| IBIS file stm32u5f9_5g9_lqfp100_dsi_smps.ibs
[IBIS ver] 4.2
[File name] stm32u5f9_5g9_lqfp100_dsi_smps.ibs
[File Rev] 1.0
[Date]  29-10-2024
[Source] Data Created at STMicroelectronics
[Notes]  File originated from ELDO simulations.
[Disclaimer]  This information is for modeling purpose only and is
   not guaranteed. The information is subject to change without
   notice.
[Copyright] Copyright 2024 STMicroelectronics Inc.
|   Component stm32u5f9_5g9_lqfp100_dsi_smps
[Component] stm32u5f9_5g9_lqfp100_dsi_smps
[Manufacturer] STMicroelectronics
[Package]
| variable   typ   min   max
R_pkg  0  NA  NA
L_pkg  0  NA  NA
C_pkg  0  NA  NA
[Pin]   signal_name   model_name
1  VBAT  power
2  PC13  io8_100m_ft_v33
3  PC14-OSC32_IN  io8_100m_ft
4  PC15-OSC32_OUT  io8_100m_ft
5  VDDDSI  nc
6  VDD11DSI  nc
7  DSI_D0P  nc
8  DSI_D0N  nc
9  VSSDSI  nc
10  DSI_CKP  nc
11  DSI_CKN  nc
12  VDD11DSI  nc
13  DSI_D1P  nc
14  DSI_D1N  nc
15  VSSDSI  nc
16  VDD  power
17  PH0-OSC_IN  io8_100m_ft
18  PH1-OSC_OUT  io8_100m_ft
19  NRST  nc
20  PC0  io8_100m_hslv_ft
21  PC1  io8_166m_hslv_i2c_ft
22  PC2  io8_100m_hslv_ft
23  PC3  io8_100m_hslv_ft
24  VSSA  nc
25  VDDA  nc
26  PA0  io8_100m_hslv_tamp_ft
27  PA1  io8_100m_hslv_tamp_ft
28  PA2  io8_100m_hslv_ft
29  PA3  io8_166m_hslv_ft
30  VSS  gnd
31  VDD  power
32  PA4  io8_100m_hslv_ft
33  PA5  io8_100m_ft
34  PA6  io8_100m_hslv_ft
35  PA7  io8_100m_hslv_ft
36  PB0  io8_100m_hslv_ft
37  PB1  io8_100m_hslv_ft
38  PB2  io8_100m_hslv_tamp_ft
39  PE7  io8_100m_hslv_ft
40  PE8  io8_100m_hslv_ft
41  PE9  io8_166m_hslv_ft
42  PE10  io8_166m_hslv_ft
43  VLXSMPS  nc
44  VDDSMPS  nc
45  VSSSMPS  nc
46  VDD11  nc
47  VSS  gnd
48  VDD  power
49  PB13  io8_100m_i2c_ft
50  PB14  io8_100m_hslv_ft
51  PB15  nc
52  PH9  io8_spi_ft
53  VSS  gnd
54  VDD  power
55  PH10  io8_spi_ft
56  PH11  io8_spi_ft
57  PH12  io8_spi_ft
58  PH13  io8_spi_ft
59  VSS  gnd
60  VDD  power
61  PH14  io8_spi_ft
62  PH15  io8_spi_ft
63  PI0  io8_spi_ft
64  PI1  io8_spi_ft
65  VSS  gnd
66  VDD  power
67  PI2  io8_spi_ft
68  PI3  io8_spi_ft
69  PA8  io8_166m_hslv_ft
70  PA9  io8_100m_usb_vbus_ft
71  PA10  io8_100m_usb_id
72  PA11  io8_100m_ft
73  PA12  io8_100m_ft
74  PA13  io8_100m_ft
75  VDDUSB  power
76  VDD  power
77  VSS  gnd
78  PA14  io8_100m_ft
79  PA15  nc
80  PC10  io8_100m_hslv_ft
81  PC11  io8_100m_hslv_ft
82  PC12  io8_166m_hslv_ft
83  PD0  io8_100m_hslv_ft
84  PD1  io8_100m_hslv_ft
85  PD2  io8_100m_hslv_ft
86  PD3  io8_166m_hslv_ft
87  PD4  io8_100m_hslv_ft
88  PD5  io8_100m_hslv_ft
89  VDD  power
90  PB3  io8_100m_hslv_ft
91  PB4  io8_100m_hslv_ft
92  PB5  io8_166m_hslv_ft
93  PB6  io8_100m_i2c_ft
94  PB7  io8_166m_hslv_i2c_ft
95  PH3-BOOT0  io8_100m_ft
96  PB8  io8_100m_hslv_ft
97  PB9  io8_100m_hslv_ft
98  VDD11  nc
99  VSS  gnd
100  VDD  power
[Package Model]   476-lqfp-14x14-100-dsi-smps-230223
[Pin Mapping]   pulldown_ref   pullup_ref   | Comment
1  nc  vsw
2  gndio  vddiom  | Depending on IO usage
| 2  gndio  vsw  | Depending on IO usage
3  gndio  vddiom  | Depending on IO usage
| 3  gndio  vsw  | Depending on IO usage
4  gndio  vddiom  | Depending on IO usage
| 4  gndio  vsw  | Depending on IO usage
5  nc  nc
6  nc  nc
7  nc  nc
8  nc  nc
9  nc  nc
10  nc  nc
11  nc  nc
12  nc  nc
13  nc  nc
14  nc  nc
15  nc  nc
16  nc  vddiom
17  gndio  vddiom
18  gndio  vddiom
19  nc  nc
20  gndio  vddiom
21  gndio  vddiom
22  gndio  vddiom
23  gndio  vddiom
24  nc  nc
25  nc  nc
26  gndio  vddiom
27  gndio  vddiom
28  gndio  vddiom
29  gndio  vddiom
30  gndio  nc
31  nc  vddiom
32  gndio  vddiom
33  gndio  vddiom
34  gndio  vddiom
35  gndio  vddiom
36  gndio  vddiom
37  gndio  vddiom
38  gndio  vddiom
39  gndio  vddiom
40  gndio  vddiom
41  gndio  vddiom
42  gndio  vddiom
43  nc  nc
44  nc  nc
45  nc  nc
46  nc  nc
47  gndio  nc
48  nc  vddiom
49  gndio  vddiom
50  gndio  vddiom
51  nc  nc
52  gndio  vddiom  | Depending on IO usage
| 52  gndio  vddhspi  | Depending on IO usage
53  gndio  nc
54  nc  vddhspi
55  gndio  vddiom
56  gndio  vddiom  | Depending on IO usage
| 56  gndio  vddhspi  | Depending on IO usage
57  gndio  vddiom  | Depending on IO usage
| 57  gndio  vddhspi  | Depending on IO usage
58  gndio  vddiom  | Depending on IO usage
| 58  gndio  vddhspi  | Depending on IO usage
59  gndio  nc
60  nc  vddhspi
61  gndio  vddiom  | Depending on IO usage
| 61  gndio  vddhspi  | Depending on IO usage
62  gndio  vddiom  | Depending on IO usage
| 62  gndio  vddhspi  | Depending on IO usage
63  gndio  vddiom  | Depending on IO usage
| 63  gndio  vddhspi  | Depending on IO usage
64  gndio  vddiom  | Depending on IO usage
| 64  gndio  vddhspi  | Depending on IO usage
65  gndio  nc
66  nc  vddhspi
67  gndio  vddiom  | Depending on IO usage
| 67  gndio  vddhspi  | Depending on IO usage
68  gndio  vddiom  | Depending on IO usage
| 68  gndio  vddhspi  | Depending on IO usage
69  gndio  vddiom
70  gndio  vddiom  | Depending on IO usage
| 70  gndio  vddusb  | Depending on IO usage
71  gndio  vddiom  | Depending on IO usage
| 71  gndio  vddusb  | Depending on IO usage
72  gndio  vddiom  | Depending on IO usage
| 72  gndio  vddusb  | Depending on IO usage
73  gndio  vddiom  | Depending on IO usage
| 73  gndio  vddusb  | Depending on IO usage
74  gndio  vddiom  | Depending on IO usage
| 74  gndio  vddusb  | Depending on IO usage
75  nc  vddusb
76  nc  vddiom
77  gndio  nc
78  gndio  vddiom
79  nc  nc
80  gndio  vddiom
81  gndio  vddiom
82  gndio  vddiom
83  gndio  vddiom
84  gndio  vddiom
85  gndio  vddiom
86  gndio  vddiom
87  gndio  vddiom
88  gndio  vddiom
89  nc  vddiom
90  gndio  vddiom
91  gndio  vddiom
92  gndio  vddiom
93  gndio  vddiom
94  gndio  vddiom
95  gndio  vddiom
96  gndio  vddiom
97  gndio  vddiom
98  nc  nc
99  gndio  nc
100  nc  vddiom
[Model Selector] io8_100m_ft
io8_100m_ft_hs_1v2  "IO8_FT 100MHz high speed @ 1.2V"
io8_100m_ft_fs_1v2  "IO8_FT 100MHz fast speed @ 1.2V"
io8_100m_ft_fs_pd_1v2  "IO8_FT 100MHz fast speed @ 1.2V pulldown"
io8_100m_ft_ms_1v2  "IO8_FT 100MHz med speed @ 1.2V"
io8_100m_ft_ms_pd_1v2  "IO8_FT 100MHz med speed @ 1.2V pulldown"
io8_100m_ft_ls_1v2  "IO8_FT 100MHz low speed @ 1.2V"
io8_100m_ft_ls_pd_1v2  "IO8_FT 100MHz low speed @ 1.2V pulldown"
io8_100m_ft_hs_1v8  "IO8_FT 100MHz high speed @ 1.8V"
io8_100m_ft_hs_pd_1v8  "IO8_FT 100MHz high speed @ 1.8V pulldown"
io8_100m_ft_fs_1v8  "IO8_FT 100MHz fast speed @ 1.8V"
io8_100m_ft_fs_pd_1v8  "IO8_FT 100MHz fast speed @ 1.8V pulldown"
io8_100m_ft_ms_1v8  "IO8_FT 100MHz med speed @ 1.8V"
io8_100m_ft_ms_pd_1v8  "IO8_FT 100MHz med speed @ 1.8V pulldown"
io8_100m_ft_ls_1v8  "IO8_FT 100MHz low speed @ 1.8V"
io8_100m_ft_ls_pd_1v8  "IO8_FT 100MHz low speed @ 1.8V pulldown"
io8_100m_ft_hs_3v3  "IO8_FT 100MHz high speed @ 3.3V"
io8_100m_ft_hs_pd_3v3  "IO8_FT 100MHz high speed @ 3.3V pulldown"
io8_100m_ft_fs_3v3  "IO8_FT 100MHz fast speed @ 3.3V"
io8_100m_ft_fs_pd_3v3  "IO8_FT 100MHz fast speed @ 3.3V pulldown"
io8_100m_ft_ms_3v3  "IO8_FT 100MHz med speed @ 3.3V"
io8_100m_ft_ms_pd_3v3  "IO8_FT 100MHz med speed @ 3.3V pulldown"
io8_100m_ft_ls_3v3  "IO8_FT 100MHz low speed @ 3.3V"
io8_100m_ft_ls_pd_3v3  "IO8_FT 100MHz low speed @ 3.3V pulldown"
[Model Selector] io8_100m_hslv_ft
io8_100m_ft_hs_1v2  "IO8_FT 100MHz high speed @ 1.2V"
io8_100m_ft_hs_pu_1v2  "IO8_FT 100MHz high speed @ 1.2V pullup"
io8_100m_ft_hs_pd_1v2  "IO8_FT 100MHz high speed @ 1.2V pulldown"
io8_100m_ft_fs_1v2  "IO8_FT 100MHz fast speed @ 1.2V"
io8_100m_ft_fs_pu_1v2  "IO8_FT 100MHz fast speed @ 1.2V pullup"
io8_100m_ft_fs_pd_1v2  "IO8_FT 100MHz fast speed @ 1.2V pulldown"
io8_100m_ft_ms_1v2  "IO8_FT 100MHz med speed @ 1.2V"
io8_100m_ft_ms_pu_1v2  "IO8_FT 100MHz med speed @ 1.2V pullup"
io8_100m_ft_ms_pd_1v2  "IO8_FT 100MHz med speed @ 1.2V pulldown"
io8_100m_ft_ls_1v2  "IO8_FT 100MHz low speed @ 1.2V"
io8_100m_ft_ls_pu_1v2  "IO8_FT 100MHz low speed @ 1.2V pullup"
io8_100m_ft_ls_pd_1v2  "IO8_FT 100MHz low speed @ 1.2V pulldown"
io8_100m_ft_hs_1v8  "IO8_FT 100MHz high speed @ 1.8V"
io8_100m_ft_hs_pu_1v8  "IO8_FT 100MHz high speed @ 1.8V pullup"
io8_100m_ft_hs_pd_1v8  "IO8_FT 100MHz high speed @ 1.8V pulldown"
io8_100m_ft_fs_1v8  "IO8_FT 100MHz fast speed @ 1.8V"
io8_100m_ft_fs_pu_1v8  "IO8_FT 100MHz fast speed @ 1.8V pullup"
io8_100m_ft_fs_pd_1v8  "IO8_FT 100MHz fast speed @ 1.8V pulldown"
io8_100m_ft_ms_1v8  "IO8_FT 100MHz med speed @ 1.8V"
io8_100m_ft_ms_pu_1v8  "IO8_FT 100MHz med speed @ 1.8V pullup"
io8_100m_ft_ms_pd_1v8  "IO8_FT 100MHz med speed @ 1.8V pulldown"
io8_100m_ft_ls_1v8  "IO8_FT 100MHz low speed @ 1.8V"
io8_100m_ft_ls_pu_1v8  "IO8_FT 100MHz low speed @ 1.8V pullup"
io8_100m_ft_ls_pd_1v8  "IO8_FT 100MHz low speed @ 1.8V pulldown"
io8_100m_ft_hs_3v3  "IO8_FT 100MHz high speed @ 3.3V"
io8_100m_ft_hs_pu_3v3  "IO8_FT 100MHz high speed @ 3.3V pullup"
io8_100m_ft_hs_pd_3v3  "IO8_FT 100MHz high speed @ 3.3V pulldown"
io8_100m_ft_fs_3v3  "IO8_FT 100MHz fast speed @ 3.3V"
io8_100m_ft_fs_pu_3v3  "IO8_FT 100MHz fast speed @ 3.3V pullup"
io8_100m_ft_fs_pd_3v3  "IO8_FT 100MHz fast speed @ 3.3V pulldown"
io8_100m_ft_ms_3v3  "IO8_FT 100MHz med speed @ 3.3V"
io8_100m_ft_ms_pu_3v3  "IO8_FT 100MHz med speed @ 3.3V pullup"
io8_100m_ft_ms_pd_3v3  "IO8_FT 100MHz med speed @ 3.3V pulldown"
io8_100m_ft_ls_3v3  "IO8_FT 100MHz low speed @ 3.3V"
io8_100m_ft_ls_pu_3v3  "IO8_FT 100MHz low speed @ 3.3V pullup"
io8_100m_ft_ls_pd_3v3  "IO8_FT 100MHz low speed @ 3.3V pulldown"
io8_100m_hslv_ft_hs_1v2  "IO8_FT 100MHz HSLV high speed @ 1.2V"
io8_100m_hslv_ft_hs_pu_1v2  "IO8_FT 100MHz HSLV high speed @ 1.2V pullup"
io8_100m_hslv_ft_hs_pd_1v2  "IO8_FT 100MHz HSLV high speed @ 1.2V pulldown"
io8_100m_hslv_ft_fs_1v2  "IO8_FT 100MHz HSLV fast speed @ 1.2V"
io8_100m_hslv_ft_fs_pu_1v2  "IO8_FT 100MHz HSLV fast speed @ 1.2V pullup"
io8_100m_hslv_ft_fs_pd_1v2  "IO8_FT 100MHz HSLV fast speed @ 1.2V pulldown"
io8_100m_hslv_ft_ms_1v2  "IO8_FT 100MHz HSLV med speed @ 1.2V"
io8_100m_hslv_ft_ms_pu_1v2  "IO8_FT 100MHz HSLV med speed @ 1.2V pullup"
io8_100m_hslv_ft_ms_pd_1v2  "IO8_FT 100MHz HSLV med speed @ 1.2V pulldown"
io8_100m_hslv_ft_ls_1v2  "IO8_FT 100MHz HSLV low speed @ 1.2V"
io8_100m_hslv_ft_ls_pu_1v2  "IO8_FT 100MHz HSLV low speed @ 1.2V pullup"
io8_100m_hslv_ft_ls_pd_1v2  "IO8_FT 100MHz HSLV low speed @ 1.2V pulldown"
io8_100m_hslv_ft_hs_1v8  "IO8_FT 100MHz HSLV high speed @ 1.8V"
io8_100m_hslv_ft_hs_pu_1v8  "IO8_FT 100MHz HSLV high speed @ 1.8V pullup"
io8_100m_hslv_ft_hs_pd_1v8  "IO8_FT 100MHz HSLV high speed @ 1.8V pulldown"
io8_100m_hslv_ft_fs_1v8  "IO8_FT 100MHz HSLV fast speed @ 1.8V"
io8_100m_hslv_ft_fs_pu_1v8  "IO8_FT 100MHz HSLV fast speed @ 1.8V pullup"
io8_100m_hslv_ft_fs_pd_1v8  "IO8_FT 100MHz HSLV fast speed @ 1.8V pulldown"
io8_100m_hslv_ft_ms_1v8  "IO8_FT 100MHz HSLV med speed @ 1.8V"
io8_100m_hslv_ft_ms_pu_1v8  "IO8_FT 100MHz HSLV med speed @ 1.8V pullup"
io8_100m_hslv_ft_ms_pd_1v8  "IO8_FT 100MHz HSLV med speed @ 1.8V pulldown"
io8_100m_hslv_ft_ls_1v8  "IO8_FT 100MHz HSLV low speed @ 1.8V"
io8_100m_hslv_ft_ls_pu_1v8  "IO8_FT 100MHz HSLV low speed @ 1.8V pullup"
io8_100m_hslv_ft_ls_pd_1v8  "IO8_FT 100MHz HSLV low speed @ 1.8V pulldown"
io8_100m_hslv_ft_hs_2v5  "IO8_FT 100MHz HSLV high speed @ 2.5V"
io8_100m_hslv_ft_hs_pu_2v5  "IO8_FT 100MHz HSLV high speed @ 2.5V pullup"
io8_100m_hslv_ft_hs_pd_2v5  "IO8_FT 100MHz HSLV high speed @ 2.5V pulldown"
io8_100m_hslv_ft_fs_2v5  "IO8_FT 100MHz HSLV fast speed @ 2.5V"
io8_100m_hslv_ft_fs_pu_2v5  "IO8_FT 100MHz HSLV fast speed @ 2.5V pullup"
io8_100m_hslv_ft_fs_pd_2v5  "IO8_FT 100MHz HSLV fast speed @ 2.5V pulldown"
io8_100m_hslv_ft_ms_2v5  "IO8_FT 100MHz HSLV med speed @ 2.5V"
io8_100m_hslv_ft_ms_pu_2v5  "IO8_FT 100MHz HSLV med speed @ 2.5V pullup"
io8_100m_hslv_ft_ms_pd_2v5  "IO8_FT 100MHz HSLV med speed @ 2.5V pulldown"
io8_100m_hslv_ft_ls_2v5  "IO8_FT 100MHz HSLV low speed @ 2.5V"
io8_100m_hslv_ft_ls_pu_2v5  "IO8_FT 100MHz HSLV low speed @ 2.5V pullup"
io8_100m_hslv_ft_ls_pd_2v5  "IO8_FT 100MHz HSLV low speed @ 2.5V pulldown"
[Model Selector] io8_100m_hslv_tamp_ft
io8_100m_ft_hs_1v2  "IO8_FT 100MHz high speed @ 1.2V"
io8_100m_ft_hs_pu_1v2  "IO8_FT 100MHz high speed @ 1.2V pullup"
io8_100m_ft_hs_pd_1v2  "IO8_FT 100MHz high speed @ 1.2V pulldown"
io8_100m_ft_fs_1v2  "IO8_FT 100MHz fast speed @ 1.2V"
io8_100m_ft_fs_pu_1v2  "IO8_FT 100MHz fast speed @ 1.2V pullup"
io8_100m_ft_fs_pd_1v2  "IO8_FT 100MHz fast speed @ 1.2V pulldown"
io8_100m_ft_ms_1v2  "IO8_FT 100MHz med speed @ 1.2V"
io8_100m_ft_ms_pu_1v2  "IO8_FT 100MHz med speed @ 1.2V pullup"
io8_100m_ft_ms_pd_1v2  "IO8_FT 100MHz med speed @ 1.2V pulldown"
io8_100m_ft_ls_1v2  "IO8_FT 100MHz low speed @ 1.2V"
io8_100m_ft_ls_pu_1v2  "IO8_FT 100MHz low speed @ 1.2V pullup"
io8_100m_ft_ls_pd_1v2  "IO8_FT 100MHz low speed @ 1.2V pulldown"
io8_100m_ft_hs_1v8  "IO8_FT 100MHz high speed @ 1.8V"
io8_100m_ft_hs_pu_1v8  "IO8_FT 100MHz high speed @ 1.8V pullup"
io8_100m_ft_hs_pd_1v8  "IO8_FT 100MHz high speed @ 1.8V pulldown"
io8_100m_ft_fs_1v8  "IO8_FT 100MHz fast speed @ 1.8V"
io8_100m_ft_fs_pu_1v8  "IO8_FT 100MHz fast speed @ 1.8V pullup"
io8_100m_ft_fs_pd_1v8  "IO8_FT 100MHz fast speed @ 1.8V pulldown"
io8_100m_ft_ms_1v8  "IO8_FT 100MHz med speed @ 1.8V"
io8_100m_ft_ms_pu_1v8  "IO8_FT 100MHz med speed @ 1.8V pullup"
io8_100m_ft_ms_pd_1v8  "IO8_FT 100MHz med speed @ 1.8V pulldown"
io8_100m_ft_ls_1v8  "IO8_FT 100MHz low speed @ 1.8V"
io8_100m_ft_ls_pu_1v8  "IO8_FT 100MHz low speed @ 1.8V pullup"
io8_100m_ft_ls_pd_1v8  "IO8_FT 100MHz low speed @ 1.8V pulldown"
io8_100m_ft_hs_3v3  "IO8_FT 100MHz high speed @ 3.3V"
io8_100m_ft_hs_pu_3v3  "IO8_FT 100MHz high speed @ 3.3V pullup"
io8_100m_ft_hs_pd_3v3  "IO8_FT 100MHz high speed @ 3.3V pulldown"
io8_100m_ft_fs_3v3  "IO8_FT 100MHz fast speed @ 3.3V"
io8_100m_ft_fs_pu_3v3  "IO8_FT 100MHz fast speed @ 3.3V pullup"
io8_100m_ft_fs_pd_3v3  "IO8_FT 100MHz fast speed @ 3.3V pulldown"
io8_100m_ft_ms_3v3  "IO8_FT 100MHz med speed @ 3.3V"
io8_100m_ft_ms_pu_3v3  "IO8_FT 100MHz med speed @ 3.3V pullup"
io8_100m_ft_ms_pd_3v3  "IO8_FT 100MHz med speed @ 3.3V pulldown"
io8_100m_ft_ls_3v3  "IO8_FT 100MHz low speed @ 3.3V"
io8_100m_ft_ls_pu_3v3  "IO8_FT 100MHz low speed @ 3.3V pullup"
io8_100m_ft_ls_pd_3v3  "IO8_FT 100MHz low speed @ 3.3V pulldown"
io8_100m_hslv_ft_hs_1v2  "IO8_FT 100MHz HSLV high speed @ 1.2V"
io8_100m_hslv_ft_hs_pu_1v2  "IO8_FT 100MHz HSLV high speed @ 1.2V pullup"
io8_100m_hslv_ft_hs_pd_1v2  "IO8_FT 100MHz HSLV high speed @ 1.2V pulldown"
io8_100m_hslv_ft_fs_1v2  "IO8_FT 100MHz HSLV fast speed @ 1.2V"
io8_100m_hslv_ft_fs_pu_1v2  "IO8_FT 100MHz HSLV fast speed @ 1.2V pullup"
io8_100m_hslv_ft_fs_pd_1v2  "IO8_FT 100MHz HSLV fast speed @ 1.2V pulldown"
io8_100m_hslv_ft_ms_1v2  "IO8_FT 100MHz HSLV med speed @ 1.2V"
io8_100m_hslv_ft_ms_pu_1v2  "IO8_FT 100MHz HSLV med speed @ 1.2V pullup"
io8_100m_hslv_ft_ms_pd_1v2  "IO8_FT 100MHz HSLV med speed @ 1.2V pulldown"
io8_100m_hslv_ft_ls_1v2  "IO8_FT 100MHz HSLV low speed @ 1.2V"
io8_100m_hslv_ft_ls_pu_1v2  "IO8_FT 100MHz HSLV low speed @ 1.2V pullup"
io8_100m_hslv_ft_ls_pd_1v2  "IO8_FT 100MHz HSLV low speed @ 1.2V pulldown"
io8_100m_hslv_ft_hs_1v8  "IO8_FT 100MHz HSLV high speed @ 1.8V"
io8_100m_hslv_ft_hs_pu_1v8  "IO8_FT 100MHz HSLV high speed @ 1.8V pullup"
io8_100m_hslv_ft_hs_pd_1v8  "IO8_FT 100MHz HSLV high speed @ 1.8V pulldown"
io8_100m_hslv_ft_fs_1v8  "IO8_FT 100MHz HSLV fast speed @ 1.8V"
io8_100m_hslv_ft_fs_pu_1v8  "IO8_FT 100MHz HSLV fast speed @ 1.8V pullup"
io8_100m_hslv_ft_fs_pd_1v8  "IO8_FT 100MHz HSLV fast speed @ 1.8V pulldown"
io8_100m_hslv_ft_ms_1v8  "IO8_FT 100MHz HSLV med speed @ 1.8V"
io8_100m_hslv_ft_ms_pu_1v8  "IO8_FT 100MHz HSLV med speed @ 1.8V pullup"
io8_100m_hslv_ft_ms_pd_1v8  "IO8_FT 100MHz HSLV med speed @ 1.8V pulldown"
io8_100m_hslv_ft_ls_1v8  "IO8_FT 100MHz HSLV low speed @ 1.8V"
io8_100m_hslv_ft_ls_pu_1v8  "IO8_FT 100MHz HSLV low speed @ 1.8V pullup"
io8_100m_hslv_ft_ls_pd_1v8  "IO8_FT 100MHz HSLV low speed @ 1.8V pulldown"
io8_100m_hslv_ft_hs_2v5  "IO8_FT 100MHz HSLV high speed @ 2.5V"
io8_100m_hslv_ft_hs_pu_2v5  "IO8_FT 100MHz HSLV high speed @ 2.5V pullup"
io8_100m_hslv_ft_hs_pd_2v5  "IO8_FT 100MHz HSLV high speed @ 2.5V pulldown"
io8_100m_hslv_ft_fs_2v5  "IO8_FT 100MHz HSLV fast speed @ 2.5V"
io8_100m_hslv_ft_fs_pu_2v5  "IO8_FT 100MHz HSLV fast speed @ 2.5V pullup"
io8_100m_hslv_ft_fs_pd_2v5  "IO8_FT 100MHz HSLV fast speed @ 2.5V pulldown"
io8_100m_hslv_ft_ms_2v5  "IO8_FT 100MHz HSLV med speed @ 2.5V"
io8_100m_hslv_ft_ms_pu_2v5  "IO8_FT 100MHz HSLV med speed @ 2.5V pullup"
io8_100m_hslv_ft_ms_pd_2v5  "IO8_FT 100MHz HSLV med speed @ 2.5V pulldown"
io8_100m_hslv_ft_ls_2v5  "IO8_FT 100MHz HSLV low speed @ 2.5V"
io8_100m_hslv_ft_ls_pu_2v5  "IO8_FT 100MHz HSLV low speed @ 2.5V pullup"
io8_100m_hslv_ft_ls_pd_2v5  "IO8_FT 100MHz HSLV low speed @ 2.5V pulldown"
io8_ft_v33_hs_1v2  "IO8_FT_V33 high speed @ 1.2V"
io8_ft_v33_hs_pu_1v2  "IO8_FT_V33 high speed @ 1.2V pullup"
io8_ft_v33_hs_pd_1v2  "IO8_FT_V33 high speed @ 1.2V pulldown"
io8_ft_v33_fs_1v2  "IO8_FT_V33 fast speed @ 1.2V"
io8_ft_v33_fs_pu_1v2  "IO8_FT_V33 fast speed @ 1.2V pullup"
io8_ft_v33_fs_pd_1v2  "IO8_FT_V33 fast speed @ 1.2V pulldown"
io8_ft_v33_ms_1v2  "IO8_FT_V33 med speed @ 1.2V"
io8_ft_v33_ms_pu_1v2  "IO8_FT_V33 med speed @ 1.2V pullup"
io8_ft_v33_ms_pd_1v2  "IO8_FT_V33 med speed @ 1.2V pulldown"
io8_ft_v33_ls_1v2  "IO8_FT_V33 low speed @ 1.2V"
io8_ft_v33_ls_pu_1v2  "IO8_FT_V33 low speed @ 1.2V pullup"
io8_ft_v33_ls_pd_1v2  "IO8_FT_V33 low speed @ 1.2V pulldown"
io8_ft_v33_hs_1v8  "IO8_FT_V33 high speed @ 1.8V"
io8_ft_v33_hs_pu_1v8  "IO8_FT_V33 high speed @ 1.8V pullup"
io8_ft_v33_hs_pd_1v8  "IO8_FT_V33 high speed @ 1.8V pulldown"
io8_ft_v33_fs_1v8  "IO8_FT_V33 fast speed @ 1.8V"
io8_ft_v33_fs_pu_1v8  "IO8_FT_V33 fast speed @ 1.8V pullup"
io8_ft_v33_fs_pd_1v8  "IO8_FT_V33 fast speed @ 1.8V pulldown"
io8_ft_v33_ms_1v8  "IO8_FT_V33 med speed @ 1.8V"
io8_ft_v33_ms_pu_1v8  "IO8_FT_V33 med speed @ 1.8V pullup"
io8_ft_v33_ms_pd_1v8  "IO8_FT_V33 med speed @ 1.8V pulldown"
io8_ft_v33_ls_1v8  "IO8_FT_V33 low speed @ 1.8V"
io8_ft_v33_ls_pu_1v8  "IO8_FT_V33 low speed @ 1.8V pullup"
io8_ft_v33_ls_pd_1v8  "IO8_FT_V33 low speed @ 1.8V pulldown"
io8_ft_v33_hs_3v3  "IO8_FT_V33 high speed @ 3.3V"
io8_ft_v33_hs_pu_3v3  "IO8_FT_V33 high speed @ 3.3V pullup"
io8_ft_v33_hs_pd_3v3  "IO8_FT_V33 high speed @ 3.3V pulldown"
io8_ft_v33_fs_3v3  "IO8_FT_V33 fast speed @ 3.3V"
io8_ft_v33_fs_pu_3v3  "IO8_FT_V33 fast speed @ 3.3V pullup"
io8_ft_v33_fs_pd_3v3  "IO8_FT_V33 fast speed @ 3.3V pulldown"
io8_ft_v33_ms_3v3  "IO8_FT_V33 med speed @ 3.3V"
io8_ft_v33_ms_pu_3v3  "IO8_FT_V33 med speed @ 3.3V pullup"
io8_ft_v33_ms_pd_3v3  "IO8_FT_V33 med speed @ 3.3V pulldown"
io8_ft_v33_ls_3v3  "IO8_FT_V33 low speed @ 3.3V"
io8_ft_v33_ls_pu_3v3  "IO8_FT_V33 low speed @ 3.3V pullup"
io8_ft_v33_ls_pd_3v3  "IO8_FT_V33 low speed @ 3.3V pulldown"
[Model Selector] io8_100m_i2c_ft
io8_100m_ft_hs_1v2  "IO8_FT 100MHz high speed @ 1.2V"
io8_100m_ft_hs_pu_1v2  "IO8_FT 100MHz high speed @ 1.2V pullup"
io8_100m_ft_hs_pd_1v2  "IO8_FT 100MHz high speed @ 1.2V pulldown"
io8_100m_ft_fs_1v2  "IO8_FT 100MHz fast speed @ 1.2V"
io8_100m_ft_fs_pu_1v2  "IO8_FT 100MHz fast speed @ 1.2V pullup"
io8_100m_ft_fs_pd_1v2  "IO8_FT 100MHz fast speed @ 1.2V pulldown"
io8_100m_ft_ms_1v2  "IO8_FT 100MHz med speed @ 1.2V"
io8_100m_ft_ms_pu_1v2  "IO8_FT 100MHz med speed @ 1.2V pullup"
io8_100m_ft_ms_pd_1v2  "IO8_FT 100MHz med speed @ 1.2V pulldown"
io8_100m_ft_ls_1v2  "IO8_FT 100MHz low speed @ 1.2V"
io8_100m_ft_ls_pu_1v2  "IO8_FT 100MHz low speed @ 1.2V pullup"
io8_100m_ft_ls_pd_1v2  "IO8_FT 100MHz low speed @ 1.2V pulldown"
io8_100m_ft_hs_1v8  "IO8_FT 100MHz high speed @ 1.8V"
io8_100m_ft_hs_pu_1v8  "IO8_FT 100MHz high speed @ 1.8V pullup"
io8_100m_ft_hs_pd_1v8  "IO8_FT 100MHz high speed @ 1.8V pulldown"
io8_100m_ft_fs_1v8  "IO8_FT 100MHz fast speed @ 1.8V"
io8_100m_ft_fs_pu_1v8  "IO8_FT 100MHz fast speed @ 1.8V pullup"
io8_100m_ft_fs_pd_1v8  "IO8_FT 100MHz fast speed @ 1.8V pulldown"
io8_100m_ft_ms_1v8  "IO8_FT 100MHz med speed @ 1.8V"
io8_100m_ft_ms_pu_1v8  "IO8_FT 100MHz med speed @ 1.8V pullup"
io8_100m_ft_ms_pd_1v8  "IO8_FT 100MHz med speed @ 1.8V pulldown"
io8_100m_ft_ls_1v8  "IO8_FT 100MHz low speed @ 1.8V"
io8_100m_ft_ls_pu_1v8  "IO8_FT 100MHz low speed @ 1.8V pullup"
io8_100m_ft_ls_pd_1v8  "IO8_FT 100MHz low speed @ 1.8V pulldown"
io8_100m_ft_hs_3v3  "IO8_FT 100MHz high speed @ 3.3V"
io8_100m_ft_hs_pu_3v3  "IO8_FT 100MHz high speed @ 3.3V pullup"
io8_100m_ft_hs_pd_3v3  "IO8_FT 100MHz high speed @ 3.3V pulldown"
io8_100m_ft_fs_3v3  "IO8_FT 100MHz fast speed @ 3.3V"
io8_100m_ft_fs_pu_3v3  "IO8_FT 100MHz fast speed @ 3.3V pullup"
io8_100m_ft_fs_pd_3v3  "IO8_FT 100MHz fast speed @ 3.3V pulldown"
io8_100m_ft_ms_3v3  "IO8_FT 100MHz med speed @ 3.3V"
io8_100m_ft_ms_pu_3v3  "IO8_FT 100MHz med speed @ 3.3V pullup"
io8_100m_ft_ms_pd_3v3  "IO8_FT 100MHz med speed @ 3.3V pulldown"
io8_100m_ft_ls_3v3  "IO8_FT 100MHz low speed @ 3.3V"
io8_100m_ft_ls_pu_3v3  "IO8_FT 100MHz low speed @ 3.3V pullup"
io8_100m_ft_ls_pd_3v3  "IO8_FT 100MHz low speed @ 3.3V pulldown"
io8_100m_i2c_ft_1v2  "IO8_FT 100MHz I2C @ 1.2V"
io8_100m_i2c_ft_pu_1v2  "IO8_FT 100MHz I2C @ 1.2V pullup"
io8_100m_i2c_ft_pd_1v2  "IO8_FT 100MHz I2C @ 1.2V pulldown"
io8_100m_i2c_ft_1v8  "IO8_FT 100MHz I2C @ 1.8V"
io8_100m_i2c_ft_pu_1v8  "IO8_FT 100MHz I2C @ 1.8V pullup"
io8_100m_i2c_ft_pd_1v8  "IO8_FT 100MHz I2C @ 1,8V pulldown"
io8_100m_i2c_ft_3v3  "IO8_FT 100MHz I2C @ 3.3V"
io8_100m_i2c_ft_pu_3v3  "IO8_FT 100MHz I2C HSLV @ 3.3V pullup"
io8_100m_i2c_ft_pd_3v3  "IO8_FT 100MHz I2C @ 3.3V pulldown"
[Model Selector] io8_100m_usb_id
io8_100m_ft_hs_1v2  "IO8_FT 100MHz high speed @ 1.2V"
io8_100m_ft_hs_pu_1v2  "IO8_FT 100MHz high speed @ 1.2V pullup"
io8_100m_ft_hs_pd_1v2  "IO8_FT 100MHz high speed @ 1.2V pulldown"
io8_100m_ft_fs_1v2  "IO8_FT 100MHz fast speed @ 1.2V"
io8_100m_ft_fs_pu_1v2  "IO8_FT 100MHz fast speed @ 1.2V pullup"
io8_100m_ft_fs_pd_1v2  "IO8_FT 100MHz fast speed @ 1.2V pulldown"
io8_100m_ft_ms_1v2  "IO8_FT 100MHz med speed @ 1.2V"
io8_100m_ft_ms_pu_1v2  "IO8_FT 100MHz med speed @ 1.2V pullup"
io8_100m_ft_ms_pd_1v2  "IO8_FT 100MHz med speed @ 1.2V pulldown"
io8_100m_ft_ls_1v2  "IO8_FT 100MHz low speed @ 1.2V"
io8_100m_ft_ls_pu_1v2  "IO8_FT 100MHz low speed @ 1.2V pullup"
io8_100m_ft_ls_pd_1v2  "IO8_FT 100MHz low speed @ 1.2V pulldown"
io8_100m_ft_hs_1v8  "IO8_FT 100MHz high speed @ 1.8V"
io8_100m_ft_hs_pu_1v8  "IO8_FT 100MHz high speed @ 1.8V pullup"
io8_100m_ft_hs_pd_1v8  "IO8_FT 100MHz high speed @ 1.8V pulldown"
io8_100m_ft_fs_1v8  "IO8_FT 100MHz fast speed @ 1.8V"
io8_100m_ft_fs_pu_1v8  "IO8_FT 100MHz fast speed @ 1.8V pullup"
io8_100m_ft_fs_pd_1v8  "IO8_FT 100MHz fast speed @ 1.8V pulldown"
io8_100m_ft_ms_1v8  "IO8_FT 100MHz med speed @ 1.8V"
io8_100m_ft_ms_pu_1v8  "IO8_FT 100MHz med speed @ 1.8V pullup"
io8_100m_ft_ms_pd_1v8  "IO8_FT 100MHz med speed @ 1.8V pulldown"
io8_100m_ft_ls_1v8  "IO8_FT 100MHz low speed @ 1.8V"
io8_100m_ft_ls_pu_1v8  "IO8_FT 100MHz low speed @ 1.8V pullup"
io8_100m_ft_ls_pd_1v8  "IO8_FT 100MHz low speed @ 1.8V pulldown"
io8_100m_ft_hs_3v3  "IO8_FT 100MHz high speed @ 3.3V"
io8_100m_ft_hs_pu_3v3  "IO8_FT 100MHz high speed @ 3.3V pullup"
io8_100m_ft_hs_pd_3v3  "IO8_FT 100MHz high speed @ 3.3V pulldown"
io8_100m_ft_fs_3v3  "IO8_FT 100MHz fast speed @ 3.3V"
io8_100m_ft_fs_pu_3v3  "IO8_FT 100MHz fast speed @ 3.3V pullup"
io8_100m_ft_fs_pd_3v3  "IO8_FT 100MHz fast speed @ 3.3V pulldown"
io8_100m_ft_ms_3v3  "IO8_FT 100MHz med speed @ 3.3V"
io8_100m_ft_ms_pu_3v3  "IO8_FT 100MHz med speed @ 3.3V pullup"
io8_100m_ft_ms_pd_3v3  "IO8_FT 100MHz med speed @ 3.3V pulldown"
io8_100m_ft_ls_3v3  "IO8_FT 100MHz low speed @ 3.3V"
io8_100m_ft_ls_pu_3v3  "IO8_FT 100MHz low speed @ 3.3V pullup"
io8_100m_ft_ls_pd_3v3  "IO8_FT 100MHz low speed @ 3.3V pulldown"
io8usb_id_nopu  "IOUSB ID @ 3.3V"
io8usb_id_pu  "IOUSB ID @ 3.3V pullup"
[Model Selector] io8_100m_usb_vbus_ft
io8_100m_ft_hs_1v2  "IO8_FT 100MHz high speed @ 1.2V"
io8_100m_ft_hs_pu_1v2  "IO8_FT 100MHz high speed @ 1.2V pullup"
io8_100m_ft_hs_pd_1v2  "IO8_FT 100MHz high speed @ 1.2V pulldown"
io8_100m_ft_fs_1v2  "IO8_FT 100MHz fast speed @ 1.2V"
io8_100m_ft_fs_pu_1v2  "IO8_FT 100MHz fast speed @ 1.2V pullup"
io8_100m_ft_fs_pd_1v2  "IO8_FT 100MHz fast speed @ 1.2V pulldown"
io8_100m_ft_ms_1v2  "IO8_FT 100MHz med speed @ 1.2V"
io8_100m_ft_ms_pu_1v2  "IO8_FT 100MHz med speed @ 1.2V pullup"
io8_100m_ft_ms_pd_1v2  "IO8_FT 100MHz med speed @ 1.2V pulldown"
io8_100m_ft_ls_1v2  "IO8_FT 100MHz low speed @ 1.2V"
io8_100m_ft_ls_pu_1v2  "IO8_FT 100MHz low speed @ 1.2V pullup"
io8_100m_ft_ls_pd_1v2  "IO8_FT 100MHz low speed @ 1.2V pulldown"
io8_100m_ft_hs_1v8  "IO8_FT 100MHz high speed @ 1.8V"
io8_100m_ft_hs_pu_1v8  "IO8_FT 100MHz high speed @ 1.8V pullup"
io8_100m_ft_hs_pd_1v8  "IO8_FT 100MHz high speed @ 1.8V pulldown"
io8_100m_ft_fs_1v8  "IO8_FT 100MHz fast speed @ 1.8V"
io8_100m_ft_fs_pu_1v8  "IO8_FT 100MHz fast speed @ 1.8V pullup"
io8_100m_ft_fs_pd_1v8  "IO8_FT 100MHz fast speed @ 1.8V pulldown"
io8_100m_ft_ms_1v8  "IO8_FT 100MHz med speed @ 1.8V"
io8_100m_ft_ms_pu_1v8  "IO8_FT 100MHz med speed @ 1.8V pullup"
io8_100m_ft_ms_pd_1v8  "IO8_FT 100MHz med speed @ 1.8V pulldown"
io8_100m_ft_ls_1v8  "IO8_FT 100MHz low speed @ 1.8V"
io8_100m_ft_ls_pu_1v8  "IO8_FT 100MHz low speed @ 1.8V pullup"
io8_100m_ft_ls_pd_1v8  "IO8_FT 100MHz low speed @ 1.8V pulldown"
io8_100m_ft_hs_3v3  "IO8_FT 100MHz high speed @ 3.3V"
io8_100m_ft_hs_pu_3v3  "IO8_FT 100MHz high speed @ 3.3V pullup"
io8_100m_ft_hs_pd_3v3  "IO8_FT 100MHz high speed @ 3.3V pulldown"
io8_100m_ft_fs_3v3  "IO8_FT 100MHz fast speed @ 3.3V"
io8_100m_ft_fs_pu_3v3  "IO8_FT 100MHz fast speed @ 3.3V pullup"
io8_100m_ft_fs_pd_3v3  "IO8_FT 100MHz fast speed @ 3.3V pulldown"
io8_100m_ft_ms_3v3  "IO8_FT 100MHz med speed @ 3.3V"
io8_100m_ft_ms_pu_3v3  "IO8_FT 100MHz med speed @ 3.3V pullup"
io8_100m_ft_ms_pd_3v3  "IO8_FT 100MHz med speed @ 3.3V pulldown"
io8_100m_ft_ls_3v3  "IO8_FT 100MHz low speed @ 3.3V"
io8_100m_ft_ls_pu_3v3  "IO8_FT 100MHz low speed @ 3.3V pullup"
io8_100m_ft_ls_pd_3v3  "IO8_FT 100MHz low speed @ 3.3V pulldown"
io8usb_adp "IOUSB ADP @ 3.3V"
io8usb_vbus "IOUSB VBUS @ 3.3V"
[Model Selector] io8_166m_hslv_ft
io8_166m_ft_hs_1v2  "IO8_FT 166MHz high speed @ 1.2V"
io8_166m_ft_hs_pu_1v2  "IO8_FT 166MHz high speed @ 1.2V pullup"
io8_166m_ft_hs_pd_1v2  "IO8_FT 166MHz high speed @ 1.2V pulldown"
io8_166m_ft_fs_1v2  "IO8_FT 166MHz fast speed @ 1.2V"
io8_166m_ft_fs_pu_1v2  "IO8_FT 166MHz fast speed @ 1.2V pullup"
io8_166m_ft_fs_pd_1v2  "IO8_FT 166MHz fast speed @ 1.2V pulldown"
io8_166m_ft_ms_1v2  "IO8_FT 166MHz med speed @ 1.2V"
io8_166m_ft_ms_pu_1v2  "IO8_FT 166MHz med speed @ 1.2V pullup"
io8_166m_ft_ms_pd_1v2  "IO8_FT 166MHz med speed @ 1.2V pulldown"
io8_166m_ft_ls_1v2  "IO8_FT 166MHz low speed @ 1.2V"
io8_166m_ft_ls_pu_1v2  "IO8_FT 166MHz low speed @ 1.2V pullup"
io8_166m_ft_ls_pd_1v2  "IO8_FT 166MHz low speed @ 1.2V pulldown"
io8_166m_ft_hs_1v8  "IO8_FT 166MHz high speed @ 1.8V"
io8_166m_ft_hs_pu_1v8  "IO8_FT 166MHz high speed @ 1.8V pullup"
io8_166m_ft_hs_pd_1v8  "IO8_FT 166MHz high speed @ 1.8V pulldown"
io8_166m_ft_fs_1v8  "IO8_FT 166MHz fast speed @ 1.8V"
io8_166m_ft_fs_pu_1v8  "IO8_FT 166MHz fast speed @ 1.8V pullup"
io8_166m_ft_fs_pd_1v8  "IO8_FT 166MHz fast speed @ 1.8V pulldown"
io8_166m_ft_ms_1v8  "IO8_FT 166MHz med speed @ 1.8V"
io8_166m_ft_ms_pu_1v8  "IO8_FT 166MHz med speed @ 1.8V pullup"
io8_166m_ft_ms_pd_1v8  "IO8_FT 166MHz med speed @ 1.8V pulldown"
io8_166m_ft_ls_1v8  "IO8_FT 166MHz low speed @ 1.8V"
io8_166m_ft_ls_pu_1v8  "IO8_FT 166MHz low speed @ 1.8V pullup"
io8_166m_ft_ls_pd_1v8  "IO8_FT 166MHz low speed @ 1.8V pulldown"
io8_166m_ft_hs_3v3  "IO8_FT 166MHz high speed @ 3.3V"
io8_166m_ft_hs_pu_3v3  "IO8_FT 166MHz high speed @ 3.3V pullup"
io8_166m_ft_hs_pd_3v3  "IO8_FT 166MHz high speed @ 3.3V pulldown"
io8_166m_ft_fs_3v3  "IO8_FT 166MHz fast speed @ 3.3V"
io8_166m_ft_fs_pu_3v3  "IO8_FT 166MHz fast speed @ 3.3V pullup"
io8_166m_ft_fs_pd_3v3  "IO8_FT 166MHz fast speed @ 3.3V pulldown"
io8_166m_ft_ms_3v3  "IO8_FT 166MHz med speed @ 3.3V"
io8_166m_ft_ms_pu_3v3  "IO8_FT 166MHz med speed @ 3.3V pullup"
io8_166m_ft_ms_pd_3v3  "IO8_FT 166MHz med speed @ 3.3V pulldown"
io8_166m_ft_ls_3v3  "IO8_FT 166MHz low speed @ 3.3V"
io8_166m_ft_ls_pu_3v3  "IO8_FT 166MHz low speed @ 3.3V pullup"
io8_166m_ft_ls_pd_3v3  "IO8_FT 166MHz low speed @ 3.3V pulldown"
io8_166m_hslv_ft_hs_1v2  "IO8_FT 166MHz HSLV high speed @ 1.2V"
io8_166m_hslv_ft_hs_pu_1v2  "IO8_FT 166MHz HSLV high speed @ 1.2V pullup"
io8_166m_hslv_ft_hs_pd_1v2  "IO8_FT 166MHz HSLV high speed @ 1.2V pulldown"
io8_166m_hslv_ft_fs_1v2  "IO8_FT 166MHz HSLV fast speed @ 1.2V"
io8_166m_hslv_ft_fs_pu_1v2  "IO8_FT 166MHz HSLV fast speed @ 1.2V pullup"
io8_166m_hslv_ft_fs_pd_1v2  "IO8_FT 166MHz HSLV fast speed @ 1.2V pulldown"
io8_166m_hslv_ft_ms_1v2  "IO8_FT 166MHz HSLV med speed @ 1.2V"
io8_166m_hslv_ft_ms_pu_1v2  "IO8_FT 166MHz HSLV med speed @ 1.2V pullup"
io8_166m_hslv_ft_ms_pd_1v2  "IO8_FT 166MHz HSLV med speed @ 1.2V pulldown"
io8_166m_hslv_ft_ls_1v2  "IO8_FT 166MHz HSLV low speed @ 1.2V"
io8_166m_hslv_ft_ls_pu_1v2  "IO8_FT 166MHz HSLV low speed @ 1.2V pullup"
io8_166m_hslv_ft_ls_pd_1v2  "IO8_FT 166MHz HSLV low speed @ 1.2V pulldown"
io8_166m_hslv_ft_hs_1v8  "IO8_FT 166MHz HSLV high speed @ 1.8V"
io8_166m_hslv_ft_hs_pu_1v8  "IO8_FT 166MHz HSLV high speed @ 1.8V pullup"
io8_166m_hslv_ft_hs_pd_1v8  "IO8_FT 166MHz HSLV high speed @ 1.8V pulldown"
io8_166m_hslv_ft_fs_1v8  "IO8_FT 166MHz HSLV fast speed @ 1.8V"
io8_166m_hslv_ft_fs_pu_1v8  "IO8_FT 166MHz HSLV fast speed @ 1.8V pullup"
io8_166m_hslv_ft_fs_pd_1v8  "IO8_FT 166MHz HSLV fast speed @ 1.8V pulldown"
io8_166m_hslv_ft_ms_1v8  "IO8_FT 166MHz HSLV med speed @ 1.8V"
io8_166m_hslv_ft_ms_pu_1v8  "IO8_FT 166MHz HSLV med speed @ 1.8V pullup"
io8_166m_hslv_ft_ms_pd_1v8  "IO8_FT 166MHz HSLV med speed @ 1.8V pulldown"
io8_166m_hslv_ft_ls_1v8  "IO8_FT 166MHz HSLV low speed @ 1.8V"
io8_166m_hslv_ft_ls_pu_1v8  "IO8_FT 166MHz HSLV low speed @ 1.8V pullup"
io8_166m_hslv_ft_ls_pd_1v8  "IO8_FT 166MHz HSLV low speed @ 1.8V pulldown"
io8_166m_hslv_ft_hs_2v5  "IO8_FT 166MHz HSLV high speed @ 2.5V"
io8_166m_hslv_ft_hs_pu_2v5  "IO8_FT 166MHz HSLV high speed @ 2.5V pullup"
io8_166m_hslv_ft_hs_pd_2v5  "IO8_FT 166MHz HSLV high speed @ 2.5V pulldown"
io8_166m_hslv_ft_fs_2v5  "IO8_FT 166MHz HSLV fast speed @ 2.5V"
io8_166m_hslv_ft_fs_pu_2v5  "IO8_FT 166MHz HSLV fast speed @ 2.5V pullup"
io8_166m_hslv_ft_fs_pd_2v5  "IO8_FT 166MHz HSLV fast speed @ 2.5V pulldown"
io8_166m_hslv_ft_ms_2v5  "IO8_FT 166MHz HSLV med speed @ 2.5V"
io8_166m_hslv_ft_ms_pu_2v5  "IO8_FT 166MHz HSLV med speed @ 2.5V pullup"
io8_166m_hslv_ft_ms_pd_2v5  "IO8_FT 166MHz HSLV med speed @ 2.5V pulldown"
io8_166m_hslv_ft_ls_2v5  "IO8_FT 166MHz HSLV low speed @ 2.5V"
io8_166m_hslv_ft_ls_pu_2v5  "IO8_FT 166MHz HSLV low speed @ 2.5V pullup"
io8_166m_hslv_ft_ls_pd_2v5  "IO8_FT 166MHz HSLV low speed @ 2.5V pulldown"
[Model Selector] io8_166m_hslv_i2c_ft
io8_166m_ft_hs_1v2  "IO8_FT 166MHz high speed @ 1.2V"
io8_166m_ft_hs_pu_1v2  "IO8_FT 166MHz high speed @ 1.2V pullup"
io8_166m_ft_hs_pd_1v2  "IO8_FT 166MHz high speed @ 1.2V pulldown"
io8_166m_ft_fs_1v2  "IO8_FT 166MHz fast speed @ 1.2V"
io8_166m_ft_fs_pu_1v2  "IO8_FT 166MHz fast speed @ 1.2V pullup"
io8_166m_ft_fs_pd_1v2  "IO8_FT 166MHz fast speed @ 1.2V pulldown"
io8_166m_ft_ms_1v2  "IO8_FT 166MHz med speed @ 1.2V"
io8_166m_ft_ms_pu_1v2  "IO8_FT 166MHz med speed @ 1.2V pullup"
io8_166m_ft_ms_pd_1v2  "IO8_FT 166MHz med speed @ 1.2V pulldown"
io8_166m_ft_ls_1v2  "IO8_FT 166MHz low speed @ 1.2V"
io8_166m_ft_ls_pu_1v2  "IO8_FT 166MHz low speed @ 1.2V pullup"
io8_166m_ft_ls_pd_1v2  "IO8_FT 166MHz low speed @ 1.2V pulldown"
io8_166m_ft_hs_1v8  "IO8_FT 166MHz high speed @ 1.8V"
io8_166m_ft_hs_pu_1v8  "IO8_FT 166MHz high speed @ 1.8V pullup"
io8_166m_ft_hs_pd_1v8  "IO8_FT 166MHz high speed @ 1.8V pulldown"
io8_166m_ft_fs_1v8  "IO8_FT 166MHz fast speed @ 1.8V"
io8_166m_ft_fs_pu_1v8  "IO8_FT 166MHz fast speed @ 1.8V pullup"
io8_166m_ft_fs_pd_1v8  "IO8_FT 166MHz fast speed @ 1.8V pulldown"
io8_166m_ft_ms_1v8  "IO8_FT 166MHz med speed @ 1.8V"
io8_166m_ft_ms_pu_1v8  "IO8_FT 166MHz med speed @ 1.8V pullup"
io8_166m_ft_ms_pd_1v8  "IO8_FT 166MHz med speed @ 1.8V pulldown"
io8_166m_ft_ls_1v8  "IO8_FT 166MHz low speed @ 1.8V"
io8_166m_ft_ls_pu_1v8  "IO8_FT 166MHz low speed @ 1.8V pullup"
io8_166m_ft_ls_pd_1v8  "IO8_FT 166MHz low speed @ 1.8V pulldown"
io8_166m_ft_hs_3v3  "IO8_FT 166MHz high speed @ 3.3V"
io8_166m_ft_hs_pu_3v3  "IO8_FT 166MHz high speed @ 3.3V pullup"
io8_166m_ft_hs_pd_3v3  "IO8_FT 166MHz high speed @ 3.3V pulldown"
io8_166m_ft_fs_3v3  "IO8_FT 166MHz fast speed @ 3.3V"
io8_166m_ft_fs_pu_3v3  "IO8_FT 166MHz fast speed @ 3.3V pullup"
io8_166m_ft_fs_pd_3v3  "IO8_FT 166MHz fast speed @ 3.3V pulldown"
io8_166m_ft_ms_3v3  "IO8_FT 166MHz med speed @ 3.3V"
io8_166m_ft_ms_pu_3v3  "IO8_FT 166MHz med speed @ 3.3V pullup"
io8_166m_ft_ms_pd_3v3  "IO8_FT 166MHz med speed @ 3.3V pulldown"
io8_166m_ft_ls_3v3  "IO8_FT 166MHz low speed @ 3.3V"
io8_166m_ft_ls_pu_3v3  "IO8_FT 166MHz low speed @ 3.3V pullup"
io8_166m_ft_ls_pd_3v3  "IO8_FT 166MHz low speed @ 3.3V pulldown"
io8_166m_hslv_ft_hs_1v2  "IO8_FT 166MHz HSLV high speed @ 1.2V"
io8_166m_hslv_ft_hs_pu_1v2  "IO8_FT 166MHz HSLV high speed @ 1.2V pullup"
io8_166m_hslv_ft_hs_pd_1v2  "IO8_FT 166MHz HSLV high speed @ 1.2V pulldown"
io8_166m_hslv_ft_fs_1v2  "IO8_FT 166MHz HSLV fast speed @ 1.2V"
io8_166m_hslv_ft_fs_pu_1v2  "IO8_FT 166MHz HSLV fast speed @ 1.2V pullup"
io8_166m_hslv_ft_fs_pd_1v2  "IO8_FT 166MHz HSLV fast speed @ 1.2V pulldown"
io8_166m_hslv_ft_ms_1v2  "IO8_FT 166MHz HSLV med speed @ 1.2V"
io8_166m_hslv_ft_ms_pu_1v2  "IO8_FT 166MHz HSLV med speed @ 1.2V pullup"
io8_166m_hslv_ft_ms_pd_1v2  "IO8_FT 166MHz HSLV med speed @ 1.2V pulldown"
io8_166m_hslv_ft_ls_1v2  "IO8_FT 166MHz HSLV low speed @ 1.2V"
io8_166m_hslv_ft_ls_pu_1v2  "IO8_FT 166MHz HSLV low speed @ 1.2V pullup"
io8_166m_hslv_ft_ls_pd_1v2  "IO8_FT 166MHz HSLV low speed @ 1.2V pulldown"
io8_166m_hslv_ft_hs_1v8  "IO8_FT 166MHz HSLV high speed @ 1.8V"
io8_166m_hslv_ft_hs_pu_1v8  "IO8_FT 166MHz HSLV high speed @ 1.8V pullup"
io8_166m_hslv_ft_hs_pd_1v8  "IO8_FT 166MHz HSLV high speed @ 1.8V pulldown"
io8_166m_hslv_ft_fs_1v8  "IO8_FT 166MHz HSLV fast speed @ 1.8V"
io8_166m_hslv_ft_fs_pu_1v8  "IO8_FT 166MHz HSLV fast speed @ 1.8V pullup"
io8_166m_hslv_ft_fs_pd_1v8  "IO8_FT 166MHz HSLV fast speed @ 1.8V pulldown"
io8_166m_hslv_ft_ms_1v8  "IO8_FT 166MHz HSLV med speed @ 1.8V"
io8_166m_hslv_ft_ms_pu_1v8  "IO8_FT 166MHz HSLV med speed @ 1.8V pullup"
io8_166m_hslv_ft_ms_pd_1v8  "IO8_FT 166MHz HSLV med speed @ 1.8V pulldown"
io8_166m_hslv_ft_ls_1v8  "IO8_FT 166MHz HSLV low speed @ 1.8V"
io8_166m_hslv_ft_ls_pu_1v8  "IO8_FT 166MHz HSLV low speed @ 1.8V pullup"
io8_166m_hslv_ft_ls_pd_1v8  "IO8_FT 166MHz HSLV low speed @ 1.8V pulldown"
io8_166m_hslv_ft_hs_2v5  "IO8_FT 166MHz HSLV high speed @ 2.5V"
io8_166m_hslv_ft_hs_pu_2v5  "IO8_FT 166MHz HSLV high speed @ 2.5V pullup"
io8_166m_hslv_ft_hs_pd_2v5  "IO8_FT 166MHz HSLV high speed @ 2.5V pulldown"
io8_166m_hslv_ft_fs_2v5  "IO8_FT 166MHz HSLV fast speed @ 2.5V"
io8_166m_hslv_ft_fs_pu_2v5  "IO8_FT 166MHz HSLV fast speed @ 2.5V pullup"
io8_166m_hslv_ft_fs_pd_2v5  "IO8_FT 166MHz HSLV fast speed @ 2.5V pulldown"
io8_166m_hslv_ft_ms_2v5  "IO8_FT 166MHz HSLV med speed @ 2.5V"
io8_166m_hslv_ft_ms_pu_2v5  "IO8_FT 166MHz HSLV med speed @ 2.5V pullup"
io8_166m_hslv_ft_ms_pd_2v5  "IO8_FT 166MHz HSLV med speed @ 2.5V pulldown"
io8_166m_hslv_ft_ls_2v5  "IO8_FT 166MHz HSLV low speed @ 2.5V"
io8_166m_hslv_ft_ls_pu_2v5  "IO8_FT 166MHz HSLV low speed @ 2.5V pullup"
io8_166m_hslv_ft_ls_pd_2v5  "IO8_FT 166MHz HSLV low speed @ 2.5V pulldown"
io8_166m_i2c_ft_1v2  "IO8_FT 166MHz I2C @ 1.2V"
io8_166m_i2c_ft_pu_1v2  "IO8_FT 166MHz I2C @ 1.2V pullup"
io8_166m_i2c_ft_pd_1v2  "IO8_FT 166MHz I2C @ 1.2V pulldown"
io8_166m_i2c_ft_1v8  "IO8_FT 166MHz I2C @ 1.8V"
io8_166m_i2c_ft_pu_1v8  "IO8_FT 166MHz I2C @ 1.8V pullup"
io8_166m_i2c_ft_pd_1v8  "IO8_FT 166MHz I2C @ 1,8V pulldown"
io8_166m_i2c_ft_3v3  "IO8_FT 166MHz I2C @ 3.3V"
io8_166m_i2c_ft_pu_3v3  "IO8_FT 166MHz I2C HSLV @ 3.3V pullup"
io8_166m_i2c_ft_pd_3v3  "IO8_FT 166MHz I2C @ 3.3V pulldown"
[Model Selector] io8_100m_ft_v33
io8_ft_v33_hs_1v2  "IO8_FT_V33 high speed @ 1.2V"
io8_ft_v33_hs_pu_1v2  "IO8_FT_V33 high speed @ 1.2V pullup"
io8_ft_v33_hs_pd_1v2  "IO8_FT_V33 high speed @ 1.2V pulldown"
io8_ft_v33_fs_1v2  "IO8_FT_V33 fast speed @ 1.2V"
io8_ft_v33_fs_pu_1v2  "IO8_FT_V33 fast speed @ 1.2V pullup"
io8_ft_v33_fs_pd_1v2  "IO8_FT_V33 fast speed @ 1.2V pulldown"
io8_ft_v33_ms_1v2  "IO8_FT_V33 med speed @ 1.2V"
io8_ft_v33_ms_pu_1v2  "IO8_FT_V33 med speed @ 1.2V pullup"
io8_ft_v33_ms_pd_1v2  "IO8_FT_V33 med speed @ 1.2V pulldown"
io8_ft_v33_ls_1v2  "IO8_FT_V33 low speed @ 1.2V"
io8_ft_v33_ls_pu_1v2  "IO8_FT_V33 low speed @ 1.2V pullup"
io8_ft_v33_ls_pd_1v2  "IO8_FT_V33 low speed @ 1.2V pulldown"
io8_ft_v33_hs_1v8  "IO8_FT_V33 high speed @ 1.8V"
io8_ft_v33_hs_pu_1v8  "IO8_FT_V33 high speed @ 1.8V pullup"
io8_ft_v33_hs_pd_1v8  "IO8_FT_V33 high speed @ 1.8V pulldown"
io8_ft_v33_fs_1v8  "IO8_FT_V33 fast speed @ 1.8V"
io8_ft_v33_fs_pu_1v8  "IO8_FT_V33 fast speed @ 1.8V pullup"
io8_ft_v33_fs_pd_1v8  "IO8_FT_V33 fast speed @ 1.8V pulldown"
io8_ft_v33_ms_1v8  "IO8_FT_V33 med speed @ 1.8V"
io8_ft_v33_ms_pu_1v8  "IO8_FT_V33 med speed @ 1.8V pullup"
io8_ft_v33_ms_pd_1v8  "IO8_FT_V33 med speed @ 1.8V pulldown"
io8_ft_v33_ls_1v8  "IO8_FT_V33 low speed @ 1.8V"
io8_ft_v33_ls_pu_1v8  "IO8_FT_V33 low speed @ 1.8V pullup"
io8_ft_v33_ls_pd_1v8  "IO8_FT_V33 low speed @ 1.8V pulldown"
io8_ft_v33_hs_3v3  "IO8_FT_V33 high speed @ 3.3V"
io8_ft_v33_hs_pu_3v3  "IO8_FT_V33 high speed @ 3.3V pullup"
io8_ft_v33_hs_pd_3v3  "IO8_FT_V33 high speed @ 3.3V pulldown"
io8_ft_v33_fs_3v3  "IO8_FT_V33 fast speed @ 3.3V"
io8_ft_v33_fs_pu_3v3  "IO8_FT_V33 fast speed @ 3.3V pullup"
io8_ft_v33_fs_pd_3v3  "IO8_FT_V33 fast speed @ 3.3V pulldown"
io8_ft_v33_ms_3v3  "IO8_FT_V33 med speed @ 3.3V"
io8_ft_v33_ms_pu_3v3  "IO8_FT_V33 med speed @ 3.3V pullup"
io8_ft_v33_ms_pd_3v3  "IO8_FT_V33 med speed @ 3.3V pulldown"
io8_ft_v33_ls_3v3  "IO8_FT_V33 low speed @ 3.3V"
io8_ft_v33_ls_pu_3v3  "IO8_FT_V33 low speed @ 3.3V pullup"
io8_ft_v33_ls_pd_3v3  "IO8_FT_V33 low speed @ 3.3V pulldown"
[Model Selector] io8_spi_ft
io8_spi_ft_hs_1v2  "IO8_FT SPI high speed @ 1.2V"
io8_spi_ft_hs_pu_1v2  "IO8_FT SPI high speed @ 1.2V pullup"
io8_spi_ft_hs_pd_1v2  "IO8_FT SPI high speed @ 1.2V pulldown"
io8_spi_ft_fs_1v2  "IO8_FT SPI fast speed @ 1.2V"
io8_spi_ft_fs_pu_1v2  "IO8_FT SPI fast speed @ 1.2V pullup"
io8_spi_ft_fs_pd_1v2  "IO8_FT SPI fast speed @ 1.2V pulldown"
io8_spi_ft_ms_1v2  "IO8_FT SPI med speed @ 1.2V"
io8_spi_ft_ms_pu_1v2  "IO8_FT SPI med speed @ 1.2V pullup"
io8_spi_ft_ms_pd_1v2  "IO8_FT SPI med speed @ 1.2V pulldown"
io8_spi_ft_ls_1v2  "IO8_FT SPI low speed @ 1.2V"
io8_spi_ft_ls_pu_1v2  "IO8_FT SPI low speed @ 1.2V pullup"
io8_spi_ft_ls_pd_1v2  "IO8_FT SPI low speed @ 1.2V pulldown"
io8_spi_ft_hs_1v8  "IO8_FT SPI high speed @ 1.8V"
io8_spi_ft_hs_pu_1v8  "IO8_FT SPI high speed @ 1.8V pullup"
io8_spi_ft_hs_pd_1v8  "IO8_FT SPI high speed @ 1.8V pulldown"
io8_spi_ft_fs_1v8  "IO8_FT SPI fast speed @ 1.8V"
io8_spi_ft_fs_pu_1v8  "IO8_FT SPI fast speed @ 1.8V pullup"
io8_spi_ft_fs_pd_1v8  "IO8_FT SPI fast speed @ 1.8V pulldown"
io8_spi_ft_ms_1v8  "IO8_FT SPI med speed @ 1.8V"
io8_spi_ft_ms_pu_1v8  "IO8_FT SPI med speed @ 1.8V pullup"
io8_spi_ft_ms_pd_1v8  "IO8_FT SPI med speed @ 1.8V pulldown"
io8_spi_ft_ls_1v8  "IO8_FT SPI low speed @ 1.8V"
io8_spi_ft_ls_pu_1v8  "IO8_FT SPI low speed @ 1.8V pullup"
io8_spi_ft_ls_pd_1v8  "IO8_FT SPI low speed @ 1.8V pulldown"
io8_spi_ft_hs_3v3  "IO8_FT SPI high speed @ 3.3V"
io8_spi_ft_hs_pu_3v3  "IO8_FT SPI high speed @ 3.3V pullup"
io8_spi_ft_hs_pd_3v3  "IO8_FT SPI high speed @ 3.3V pulldown"
io8_spi_ft_fs_3v3  "IO8_FT SPI fast speed @ 3.3V"
io8_spi_ft_fs_pu_3v3  "IO8_FT SPI fast speed @ 3.3V pullup"
io8_spi_ft_fs_pd_3v3  "IO8_FT SPI fast speed @ 3.3V pulldown"
io8_spi_ft_ms_3v3  "IO8_FT SPI med speed @ 3.3V"
io8_spi_ft_ms_pu_3v3  "IO8_FT SPI med speed @ 1.8V pullup"
io8_spi_ft_ms_pd_3v3  "IO8_FT SPI med speed @ 3.3V pulldown"
io8_spi_ft_ls_3v3  "IO8_FT SPI low speed @ 3.3V"
io8_spi_ft_ls_pu_3v3  "IO8_FT SPI low speed @ 3.3V pullup"
io8_spi_ft_ls_pd_3v3  "IO8_FT SPI low speed @ 3.3V pulldown"
io8_spi_hslv_ft_hs_1v2  "IO8_FT SPI HSLV high speed @ 1.2V"
io8_spi_hslv_ft_hs_pu_1v2  "IO8_FT SPI HSLV high speed @ 1.2V pullup"
io8_spi_hslv_ft_hs_pd_1v2  "IO8_FT SPI HSLV high speed @ 1.2V pulldown"
io8_spi_hslv_ft_fs_1v2  "IO8_FT SPI HSLV fast speed @ 1.2V"
io8_spi_hslv_ft_fs_pu_1v2  "IO8_FT SPI HSLV fast speed @ 1.2V pullup"
io8_spi_hslv_ft_fs_pd_1v2  "IO8_FT SPI HSLV fast speed @ 1.2V pulldown"
io8_spi_hslv_ft_ms_1v2  "IO8_FT SPI HSLV med speed @ 1.2V"
io8_spi_hslv_ft_ms_pu_1v2  "IO8_FT SPI HSLV med speed @ 1.2V pullup"
io8_spi_hslv_ft_ms_pd_1v2  "IO8_FT SPI HSLV med speed @ 1.2V pulldown"
io8_spi_hslv_ft_ls_1v2  "IO8_FT SPI HSLV low speed @ 1.2V"
io8_spi_hslv_ft_ls_pu_1v2  "IO8_FT SPI HSLV low speed @ 1.2V pullup"
io8_spi_hslv_ft_ls_pd_1v2  "IO8_FT SPI HSLV low speed @ 1.2V pulldown"
io8_spi_hslv_ft_hs_1v8  "IO8_FT SPI HSLV high speed @ 1.8V"
io8_spi_hslv_ft_hs_pu_1v8  "IO8_FT SPI HSLV high speed @ 1.8V pullup"
io8_spi_hslv_ft_hs_pd_1v8  "IO8_FT SPI HSLV high speed @ 1.8V pulldown"
io8_spi_hslv_ft_fs_1v8  "IO8_FT SPI HSLV fast speed @ 1.8V"
io8_spi_hslv_ft_fs_pu_1v8  "IO8_FT SPI HSLV fast speed @ 1.8V pullup"
io8_spi_hslv_ft_fs_pd_1v8  "IO8_FT SPI HSLV fast speed @ 1.8V pulldown"
io8_spi_hslv_ft_ms_1v8  "IO8_FT SPI HSLV med speed @ 1.8V"
io8_spi_hslv_ft_ms_pu_1v8  "IO8_FT SPI HSLV med speed @ 1.8V pullup"
io8_spi_hslv_ft_ms_pd_1v8  "IO8_FT SPI HSLV med speed @ 1.8V pulldown"
io8_spi_hslv_ft_ls_1v8  "IO8_FT SPI HSLV low speed @ 1.8V"
io8_spi_hslv_ft_ls_pu_1v8  "IO8_FT SPI HSLV low speed @ 1.8V pullup"
io8_spi_hslv_ft_ls_pd_1v8  "IO8_FT SPI HSLV low speed @ 1.8V pulldown"
io8_spi_hslv_ft_hs_2v5  "IO8_FT SPI HSLV high speed @ 2.5V"
io8_spi_hslv_ft_hs_pu_2v5  "IO8_FT SPI HSLV high speed @ 2.5V pullup"
io8_spi_hslv_ft_hs_pd_2v5  "IO8_FT SPI HSLV high speed @ 2.5V pulldown"
io8_spi_hslv_ft_fs_2v5  "IO8_FT SPI HSLV fast speed @ 2.5V"
io8_spi_hslv_ft_fs_pu_2v5  "IO8_FT SPI HSLV fast speed @ 2.5V pullup"
io8_spi_hslv_ft_fs_pd_2v5  "IO8_FT SPI HSLV fast speed @ 2.5V pulldown"
io8_spi_hslv_ft_ms_2v5  "IO8_FT SPI HSLV med speed @ 2.5V"
io8_spi_hslv_ft_ms_pu_2v5  "IO8_FT SPI HSLV med speed @ 2.5V pullup"
io8_spi_hslv_ft_ms_pd_2v5  "IO8_FT SPI HSLV med speed @ 2.5V pulldown"
io8_spi_hslv_ft_ls_2v5  "IO8_FT SPI HSLV low speed @ 2.5V"
io8_spi_hslv_ft_ls_pu_2v5  "IO8_FT SPI HSLV low speed @ 2.5V pullup"
io8_spi_hslv_ft_ls_pd_2v5  "IO8_FT SPI HSLV low speed @ 2.5V pulldown"
[Define Package Model]  476-lqfp-14x14-100-dsi-smps-230223
[Manufacturer]  Unknown
[OEM]  Unknown
[Description]  None
[Number Of Pins]  97
[Pin Numbers]
| Pin Num   Terminal Name
11 | DSI_CKN
10 | DSI_CKP
8 | DSI_D0N
7 | DSI_D0P
14 | DSI_D1N
13 | DSI_D1P
19 | NRST
26 | PA0
27 | PA1
28 | PA2
29 | PA3
32 | PA4
33 | PA5
34 | PA6
35 | PA7
69 | PA8
70 | PA9
71 | PA10
72 | PA11
73 | PA12
74 | PA13
78 | PA14
79 | PA15
36 | PB0
37 | PB1
38 | PB2
90 | PB3
91 | PB4
92 | PB5
93 | PB6
94 | PB7
96 | PB8
97 | PB9
49 | PB13
50 | PB14
51 | PB15
20 | PC0
21 | PC1
22 | PC2
23 | PC3
80 | PC10
81 | PC11
82 | PC12
2 | PC13
3 | PC14-OSC32_IN
4 | PC15-OSC32_OUT
83 | PD0
84 | PD1
85 | PD2
86 | PD3
87 | PD4
88 | PD5
39 | PE7
40 | PE8
41 | PE9
42 | PE10
17 | PH0-OSC_IN
18 | PH1
95 | PH3-BOOT0
52 | PH9
55 | PH10
56 | PH11
57 | PH12
58 | PH13
61 | PH14
62 | PH15
63 | PI0
64 | PI1
67 | PI2
68 | PI3
46 | VDD11
98 | VDD11
1 | VBAT
54 | VDD
60 | VDD
66 | VDD
5 | VDDDSI
6 | VDD11DSI
12 | VDD11DSI
75 | VDDUSB
16 | VDD
31 | VDD
48 | VDD
76 | VDD
89 | VDD
100 | VDD
25 | VDDA
44 | VDDSMPS
43 | VLXSMPS
30 | VSS
9 | VSSDSI
15 | VSSDSI
53 | VSS
59 | VSS
65 | VSS
24 | VSSA
45 | VSSSMPS
|[Merged Pins]  30
|47  |  VSS
|77  |  VSS
|99  |  VSS
[Model Data]
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[End Model Data]
[End Package Model]
| Models and submodels in the file (274): io8_100m_ft_hs_1v2 (I/O), io8_100m_ft_hs_pu_1v2 (I/O), io8_100m_ft_hs_pd_1v2 (I/O), io8_100m_ft_fs_1v2 (I/O), io8_100m_ft_fs_pu_1v2 (I/O), io8_100m_ft_fs_pd_1v2 (I/O), io8_100m_ft_ms_1v2 (I/O), io8_100m_ft_ms_pu_1v2 (I/O), io8_100m_ft_ms_pd_1v2 (I/O), io8_100m_ft_ls_1v2 (I/O), io8_100m_ft_ls_pu_1v2 (I/O), io8_100m_ft_ls_pd_1v2 (I/O), io8_100m_ft_hs_1v8 (I/O), io8_100m_ft_hs_pu_1v8 (I/O), io8_100m_ft_hs_pd_1v8 (I/O), io8_100m_ft_fs_1v8 (I/O), io8_100m_ft_fs_pu_1v8 (I/O), io8_100m_ft_fs_pd_1v8 (I/O), io8_100m_ft_ms_1v8 (I/O), io8_100m_ft_ms_pu_1v8 (I/O), io8_100m_ft_ms_pd_1v8 (I/O), io8_100m_ft_ls_1v8 (I/O), io8_100m_ft_ls_pu_1v8 (I/O), io8_100m_ft_ls_pd_1v8 (I/O), io8_100m_ft_hs_3v3 (I/O), io8_100m_ft_hs_pu_3v3 (I/O), io8_100m_ft_hs_pd_3v3 (I/O), io8_100m_ft_fs_3v3 (I/O), io8_100m_ft_fs_pu_3v3 (I/O), io8_100m_ft_fs_pd_3v3 (I/O), io8_100m_ft_ms_3v3 (I/O), io8_100m_ft_ms_pu_3v3 (I/O), io8_100m_ft_ms_pd_3v3 (I/O), io8_100m_ft_ls_3v3 (I/O), io8_100m_ft_ls_pu_3v3 (I/O), io8_100m_ft_ls_pd_3v3 (I/O), io8_100m_hslv_ft_hs_1v2 (I/O), io8_100m_hslv_ft_hs_pu_1v2 (I/O), io8_100m_hslv_ft_hs_pd_1v2 (I/O), io8_100m_hslv_ft_fs_1v2 (I/O), io8_100m_hslv_ft_fs_pu_1v2 (I/O), io8_100m_hslv_ft_fs_pd_1v2 (I/O), io8_100m_hslv_ft_ms_1v2 (I/O), io8_100m_hslv_ft_ms_pu_1v2 (I/O), io8_100m_hslv_ft_ms_pd_1v2 (I/O), io8_100m_hslv_ft_ls_1v2 (I/O), io8_100m_hslv_ft_ls_pu_1v2 (I/O), io8_100m_hslv_ft_ls_pd_1v2 (I/O), io8_100m_hslv_ft_hs_1v8 (I/O), io8_100m_hslv_ft_hs_pu_1v8 (I/O), io8_100m_hslv_ft_hs_pd_1v8 (I/O), io8_100m_hslv_ft_fs_1v8 (I/O), io8_100m_hslv_ft_fs_pu_1v8 (I/O), io8_100m_hslv_ft_fs_pd_1v8 (I/O), io8_100m_hslv_ft_ms_1v8 (I/O), io8_100m_hslv_ft_ms_pu_1v8 (I/O), io8_100m_hslv_ft_ms_pd_1v8 (I/O), io8_100m_hslv_ft_ls_1v8 (I/O), io8_100m_hslv_ft_ls_pu_1v8 (I/O), io8_100m_hslv_ft_ls_pd_1v8 (I/O), io8_100m_hslv_ft_hs_2v5 (I/O), io8_100m_hslv_ft_hs_pu_2v5 (I/O), io8_100m_hslv_ft_hs_pd_2v5 (I/O), io8_100m_hslv_ft_fs_2v5 (I/O), io8_100m_hslv_ft_fs_pu_2v5 (I/O), io8_100m_hslv_ft_fs_pd_2v5 (I/O), io8_100m_hslv_ft_ms_2v5 (I/O), io8_100m_hslv_ft_ms_pu_2v5 (I/O), io8_100m_hslv_ft_ms_pd_2v5 (I/O), io8_100m_hslv_ft_ls_2v5 (I/O), io8_100m_hslv_ft_ls_pu_2v5 (I/O), io8_100m_hslv_ft_ls_pd_2v5 (I/O), io8_166m_ft_hs_1v2 (I/O), io8_166m_ft_hs_pu_1v2 (I/O), io8_166m_ft_hs_pd_1v2 (I/O), io8_166m_ft_fs_1v2 (I/O), io8_166m_ft_fs_pu_1v2 (I/O), io8_166m_ft_fs_pd_1v2 (I/O), io8_166m_ft_ms_1v2 (I/O), io8_166m_ft_ms_pu_1v2 (I/O)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
